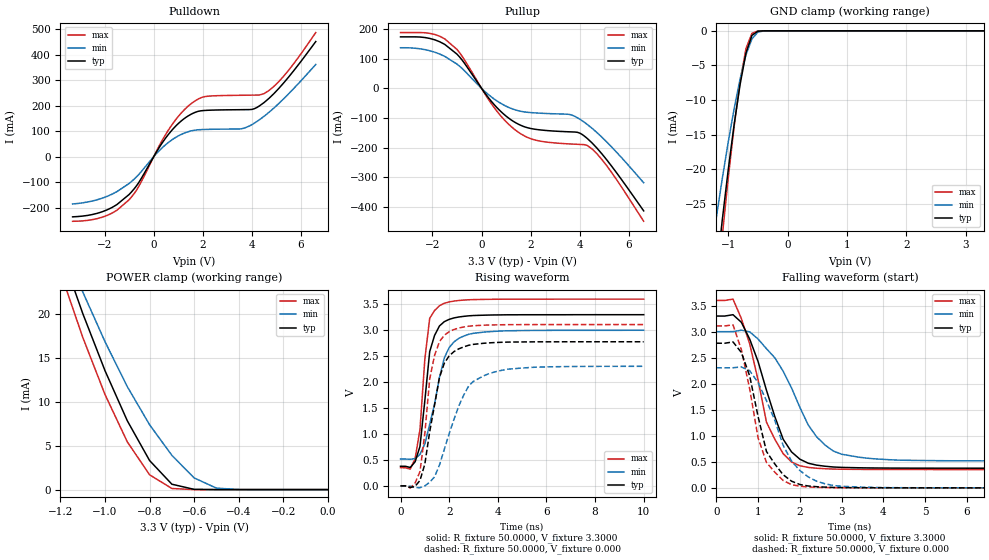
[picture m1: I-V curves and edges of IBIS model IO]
| Xilinx XC17V00 IBIS File
[IBIS ver]   2.1
[File name]   xc17v00.ibs
[File Rev]   0.2
[Date]   Aug 21, 2001
[Source]   Hspice simulations
[Notes]   Xilinx IBIS model for XC17V00 I/O
|   The package models are provided for SO20, VO8, VQ44, PC20
|   and PC44 package types, with SO20 being selected as a
|   default. Please make your own selection of the packages
|   by commenting out the unused ones.
|   COMMENTS: Models include process corners for MIN and MAX.
[Disclaimer]   The data in this model is derived from SPICE simulations
|   using modeling information extracted from the target pro-
|   cess. While a great deal of care has been take to provide
|   information that is accurate, this model is considered
|   preliminary as it has not been verified by actual silicon
|   measurement. Treat the data in this model as preliminary
|   until actual silicon verification is performed.
[Copyright]   Copyright 2001, Xilinx Inc., All rights reserved
|   Component XC17V00
|   >>> Make Your Selection of the Package type Below <<<
[Component]   XC17V00
[Manufacturer]   Xilinx Inc.
[Package]
| For package type SO20
| variable   typ   min   max
R_pkg   50.0000m   40.0000m   60.0000m
L_pkg   2.3500nH   1.7000nH   3.0000nH
C_pkg   0.3000pF   0.2000pF   0.4000pF
| For package type VO8
| variable   typ   min   max
|R_pkg   42.5000m   41.0000m   44.0000m
|L_pkg   1.8000nH   1.6000nH   2.0000nH
|C_pkg   0.3000pF   0.3000pF   0.3000pF
| For package type PC20
| variable   typ   min   max
|R_pkg   56.0000m   52.0000m   60.0000m
|L_pkg   3.3000nH   3.0000nH   3.6000nH
|C_pkg   0.7000pF   0.7000pF   0.7000pF
| For package type VQ44
| variable   typ   min   max
|R_pkg   53.0000m   46.0000m   60.0000m
|L_pkg   2.1000nH   1.8000nH   2.4000nH
|C_pkg   0.2500pF   0.2000pF   0.3000pF
| For package type PC44
| variable   typ   min   max
|R_pkg   62.5000m   56.0000m   69.0000m
|L_pkg   3.4000nH   3.1000nH   3.7000nH
|C_pkg   0.8500pF   0.7000pF   1.0000pF
[Pin]  signal_name   model_name   R_pin   L_pin   C_pin
VCC0   VCC0   POWER   NA   NA   NA
PGND   GND   GND   NA   NA   NA
io   io   IO   NA   NA   NA
| Models and submodels in the file (1): IO (I/O)
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|   Model IO
[Model]   IO
Model_type   I/O
Polarity   Non-Inverting
Enable   Active-Low
Vinl =   0.8000V
Vinh =   2.0000V
Vmeas =   1.6500V
Cref =  50.0000pF
Rref =   1.0000M
Vref =  0.000V
C_comp   18.4570pF   15.2520pF   21.6610pF
[Temperature Range]   25.0000   100.0000   0.000
[Voltage Range]   3.3000V   3.0000V   3.6000V
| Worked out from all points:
|   slope of the pulldown table from 0 to 0.495 V, typ, clamps not added: 6.66 ohm
|   slope of the pullup table from 0 to 0.495 V, typ, clamps not added: 9.33 ohm
|   GND clamp passes 1 mA (typ) near -0.61 V on its own axis
|   POWER clamp passes 1 mA (typ) near -0.71 V on its own axis
|   rising waveform, R_fixture 50.0000, V_fixture 3.3000: 20-80 % time 436ps typ, 730ps min, 359ps max; typ from 0.377 V to 3.3 V
|   rising waveform, R_fixture 50.0000, V_fixture 0.000: 20-80 % time 654ps typ, 1.07ns min, 494ps max; typ from 0 V to 2.78 V
|   falling waveform, R_fixture 50.0000, V_fixture 3.3000: 20-80 % time 722ps typ, 976ps min, 636ps max; typ from 3.3 V to 0.377 V
|   falling waveform, R_fixture 50.0000, V_fixture 0.000: 20-80 % time 553ps typ, 758ps min, 500ps max; typ from 2.78 V to 0 V
[Pulldown]
| voltage   I(typ)   I(min)   I(max)
-3.3V     -235.5mA   -185.1mA   -253mA
-1.9V     -208.3mA   -155.4mA   -230.1mA
-1V       -147.9mA   -104.6mA   -168.6mA
-600mV    -100.2mA   -68.8mA    -115.2mA
600mV     87.51mA    56.07mA    104.6mA
1.5V      165.5mA    100.8mA    206.1mA
2.1V      181.7mA    107.1mA    236.1mA
3.6V      184.6mA    110.2mA    241.1mA
4.2V      193mA      138mA      241.8mA
4.5V      212.9mA    159mA      247.7mA
5.1V      268.4mA    209.3mA    295.3mA
6.6V      451.6mA    361.8mA    486.9mA
[Pullup]
| voltage   I(typ)   I(min)   I(max)
-3.3V     173.7mA    137mA      188.2mA
-2.3V     171.4mA    130.6mA    187.6mA
-1.5V     148.4mA    108mA      167mA
-900mV    106.3mA    75.07mA    121mA
600mV     -62.65mA   -40.98mA   -74.34mA
1.6V      -124.8mA   -77.44mA   -153.5mA
2.3V      -139.3mA   -83.36mA   -176.6mA
3.6V      -146.7mA   -88.4mA    -187.5mA
4.1V      -155.8mA   -109.5mA   -189.4mA
4.5V      -184.2mA   -134.8mA   -204.4mA
4.9V      -221mA     -164.8mA   -240.1mA
6.6V      -413.2mA   -318.3mA   -448.4mA
[GND_clamp]
| voltage   I(typ)   I(min)   I(max)
-3.3V     -261mA     -199.2mA   -292mA
-1.3V     -43.63mA   -33.09mA   -48.56mA
-1.2V     -35.26mA   -27.06mA   -38.85mA
-1.1V     -27.42mA   -21.41mA   -29.76mA
-1V       -20.16mA   -16.14mA   -21.38mA
-900mV    -13.57mA   -11.29mA   -13.84mA
-800mV    -7.783mA   -6.972mA   -7.351mA
-700mV    -3.184mA   -3.462mA   -2.544mA
-600mV    -655.5uA   -1.163mA   -358.1uA
-500mV    -54.49uA   -187.3uA   -18.85uA
-400mV    -2.799uA   -15.67uA   -616nA
3.3V      36.78pA    508.5nA    34.99pA
[POWER_clamp]
| voltage   I(typ)   I(min)   I(max)
-3.3V     256.5mA    216.1mA    270.9mA
-1.2V     27.33mA    28.71mA    24.81mA
-1.1V     20.11mA    22.57mA    17.39mA
-1V       13.57mA    16.88mA    10.85mA
-900mV    7.856mA    11.75mA    5.449mA
-800mV    3.316mA    7.399mA    1.689mA
-700mV    615uA      3.909mA    126.2uA
-600mV    27.52uA    1.33mA     2.745uA
-500mV    838.8nA    167.1uA    53.67nA
-400mV    24.35nA    9.796uA    1.071nA
0V        37.72pA    531.1pA    39.58pA
[Ramp]
| variable   typ   min   max
dV/dt_r   1.6668/0.5680n   1.3830/1.0776n   1.8660/0.4122n
dV/dt_f   1.7536/0.6617n   1.4895/0.9663n   1.9490/0.5837n
R_load = 50.0000
[Rising Waveform]
R_fixture = 50.0000
V_fixture = 3.3000
V_fixture_min = 3.0000
V_fixture_max = 3.6000
L_fixture = 0.000H
C_fixture = 0.000F
| time   V(typ)   V(min)   V(max)
0s        377.4mV    517.5mV    351.7mV
400ps     354.7mV    512.1mV    323.5mV
600ps     464.1mV    525.9mV    523.4mV
800ps     760.1mV    605.6mV    1.087V
1ns       1.644V     810.2mV    2.443V
1.2ns     2.589V     1.188V     3.231V
1.6ns     3.082V     2.088V     3.473V
2ns       3.21V      2.666V     3.546V
2.8ns     3.278V     2.922V     3.588V
10ns      3.3V       3V         3.6V
[Rising Waveform]
R_fixture = 50.0000
V_fixture = 0.000
V_fixture_min = 0.000
V_fixture_max = 0.000
L_fixture = 0.000H
C_fixture = 0.000F
| time   V(typ)   V(min)   V(max)
0s        0V         0V         0V
400ps     -32.37mV   -6.098mV   -38.44mV
800ps     103.8mV    -35.08mV   274.1mV
1.2ns     1.045V     70.26mV    2.061V
1.4ns     1.56V      173.9mV    2.515V
1.6ns     2.087V     399.2mV    2.78V
2ns       2.506V     1.005V     2.972V
2.8ns     2.71V      1.922V     3.078V
3.6ns     2.756V     2.156V     3.1V
10ns      2.778V     2.305V     3.11V
[Falling Waveform]
R_fixture = 50.0000
V_fixture = 3.3000
V_fixture_min = 3.0000
V_fixture_max = 3.6000
L_fixture = 0.000H
C_fixture = 0.000F
| time   V(typ)   V(min)   V(max)
0s        3.3V       3V         3.6V
400ps     3.325V     3.001V     3.624V
600ps     3.18V      3.028V     3.252V
800ps     2.856V     2.996V     2.763V
1.2ns     1.877V     2.673V     1.263V
1.6ns     934.4mV    2.24V      656.9mV
2ns       550.9mV    1.546V     423.9mV
2.6ns     415.6mV    824mV      367.5mV
3.4ns     385.9mV    590.5mV    355.1mV
10ns      377.4mV    517.5mV    351.7mV
[Falling Waveform]
R_fixture = 50.0000
V_fixture = 0.000
V_fixture_min = 0.000
V_fixture_max = 0.000
L_fixture = 0.000H
C_fixture = 0.000F
| time   V(typ)   V(min)   V(max)
0s        2.778V     2.305V     3.11V
400ps     2.803V     2.307V     3.131V
600ps     2.6V       2.321V     2.656V
800ps     2.147V     2.25V      1.896V
1ns       1.37V      2.02V      962mV
1.2ns     699.6mV    1.677V     489.8mV
1.8ns     128.5mV    516.1mV    61.51mV
2.4ns     22.24mV    127.8mV    10.37mV
3ns       5.627mV    30.96mV    2.718mV
10ns      2.947uV    5.944uV    1.401uV
